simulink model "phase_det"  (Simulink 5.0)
settings: Solver=ode4  StartTime=0.0  StopTime=100  FixedStep=0.001  RelTol=1e-6

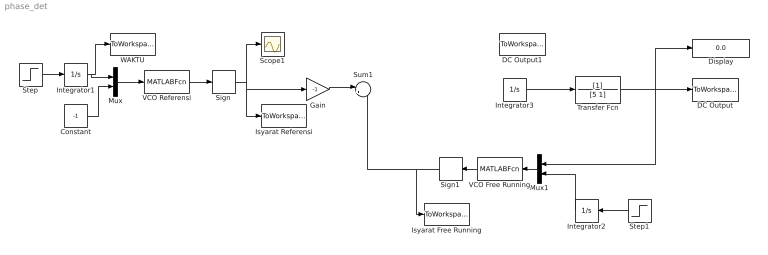
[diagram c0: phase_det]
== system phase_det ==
  Constant : Constant  Value=-1
  DC Output : ToWorkspace  VariableName=vout  SampleTime=-1  SaveFormat=Array
  DC Output1 : ToWorkspace  VariableName=outcomp  SampleTime=-1  SaveFormat=Array
  Display : Display
  Gain : Gain  Gain=-1
  Integrator1 : Integrator
  Integrator2 : Integrator  Orientation=left
  Integrator3 : Integrator
  Isyarat Free Running : ToWorkspace  VariableName=frun  SampleTime=-1  SaveFormat=Array
  Isyarat Referensi : ToWorkspace  VariableName=fref  SampleTime=-1  SaveFormat=Array
  Mux : Mux  Inputs=2
  Mux1 : Mux  Orientation=left  Inputs=2
  Scope1 : Scope
  Sign : Signum
  Sign1 : Signum  Orientation=left
  Step : Step  Time=0  SampleTime=0
  Step1 : Step  Orientation=left  Time=0  SampleTime=0
  Sum1 : Sum  Inputs=|++
  Transfer Fcn : TransferFcn  Denominator=[5 1]
  VCO Free Running : MATLABFcn  Orientation=left  MATLABFcn=vcorun
  VCO Referensi : MATLABFcn  MATLABFcn=vcoref
  WAKTU : ToWorkspace  VariableName=time  SampleTime=-1  SaveFormat=Array
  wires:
  Step/1 -> Integrator1/1
  Integrator1/1 -> Mux/1, WAKTU/1
  Mux/1 -> VCO Referensi/1
  Sign/1 -> Scope1/1, Isyarat Referensi/1, Gain/1
  Constant/1 -> Mux/2
  VCO Referensi/1 -> Sign/1
  VCO Free Running/1 -> Sign1/1
  Sign1/1 -> Isyarat Free Running/1, Sum1/2
  Mux1/1 -> VCO Free Running/1
  Step1/1 -> Integrator2/1
  Integrator2/1 -> Mux1/2
  ? -> Integrator3/1, DC Output1/1
  Sum1/1 -> ?
  Integrator3/1 -> Transfer Fcn/1
  Gain/1 -> Sum1/1
  Transfer Fcn/1 -> DC Output/1, Display/1, Mux1/1
